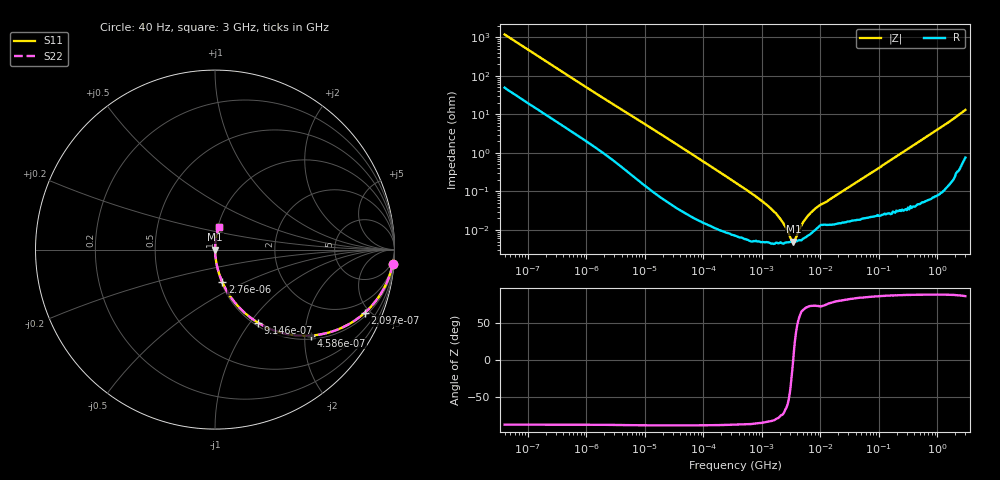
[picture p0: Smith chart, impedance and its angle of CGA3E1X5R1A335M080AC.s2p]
! S-parameter Generated by TDK Corporation
! Copyright(C) 2015 TDK Corporation.
! All Rights Reserved.
! TDK P/N: CGA3E1X5R1A335M080AC (Multilayer Ceramic Chip Capacitors)
! Property: C=3.3uF
! Size(LxWxT): 1.6x0.8x0.8mm, 0.063x0.031x0.031inches
! Model Type: s2p (Touchstone File Format Version 1.0)
! Frequency: DC=Yes Start=0.00004MHz Stop=3000MHz 396points Log-sweep
! Note: This model was converted from impedance.
! Model Generated on Jun. 23, 2015
! Hash(MD5):
! Port Assignments:
!  1 ---| |--- 2
! Applicable Conditions:
!  Temperature = 25 degC
!  DC Bias Voltage = 0 V
!  Small Signal Operation
! Terms and conditions regarding TDK Simulation Models
! (1)This simulation model is being provided solely for informational purposes. Please refer to the specifications of the products in terms of detailed characteristics of such products.
! (2)In no event shall TDK Corporation of any of its subsidiaries be liable for any loss or damage arising, directly or indirectly,
!  From any information contained in this simulation model, including, but not limited to loss or damages arising from any inaccuracies, omissions or errors in connection with such information.
! (3)Any and all copyrights on this simulation model are owned by TDK Corporation.
!  Duplication or redistribution of this simulation model without prior written permission from TDK Corporation is prohibited.
! (4)This simulation model is subject to any modification or change without any prior notice.
! (5)Neither TDK Corporation nor any of its subsidiaries shall make any warranty, express or implied,
!  Including but not limited to the correctness, implied warranties of merchantability and fitness for a particular purpose with respect to this simulation models.
! (6)The use of this simulation model shall be deemed to have consented to the terms and conditions hereof.
# MHz S MA R 50
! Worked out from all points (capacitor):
!   395 points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, 40 Hz to 3 GHz, reference 50 ohm
!   read as one part in series: C = 3.34 uF near 41.88 Hz
!   lowest |Z| = 4.99 mohm at 3.459 MHz (marker M1)
!   series resonance near 3.418 MHz, so ESL is about 650 pH
!   S11 on the Smith chart (normalised r, x): 40 Hz: 2, -24; 209.7 Hz: 1.19, -4.65; 458.6 Hz: 1.09, -2.15; 914.6 Hz: 1.04, -1.10; 2.76 kHz: 1.01, -0.38; 3 GHz: 1.02, +0.26
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4e-05  0.993 -4.8  0.08367 82.8  0.08367 82.8  0.993 -4.8
0.0001100992  0.9666 -12.7  0.2202 75.0  0.2202 75.0  0.9666 -12.7
0.000209705  0.9055 -22.9  0.3891 64.8  0.3891 64.8  0.9055 -22.9
0.0004585594  0.7187 -41.8  0.6669 45.9  0.6669 45.9  0.7187 -41.8
0.000834128  0.5054 -57.4  0.843 30.3  0.843 30.3  0.5054 -57.4
0.0009145504  0.4728 -59.5  0.8625 28.2  0.8625 28.2  0.4728 -59.5
0.001517294  0.3144 -69.5  0.9373 18.3  0.9373 18.3  0.3144 -69.5
0.002759985  0.1847 -77.3  0.9763 10.6  0.9763 10.6  0.1847 -77.3
0.006319477  0.08583 -83.4  0.9939 4.9  0.9939 4.9  0.08583 -83.4
0.01739424  0.03272 -86.8  0.9987 1.9  0.9987 1.9  0.03272 -86.8
0.3464102  0.00173 -87.6  0.9999 0.1  0.9999 0.1  0.00173 -87.6
1.315913  0.0004008 -83.3  1 0.0  1 0.0  0.0004008 -83.3
1.901634  0.0002278 -78.6  1 0.0  1 0.0  0.0002278 -78.6
2.748062  9.565e-05 -60.2  1 0.0  1 0.0  9.565e-05 -60.2
3.459106  4.994e-05 4.8  1 -0.0  1 -0.0  4.994e-05 4.8
4.354128  0.0001032 58.3  0.9999 -0.0  0.9999 -0.0  0.0001032 58.3
5.234209  0.000171 69.0  0.9999 -0.0  0.9999 -0.0  0.000171 69.0
7.22376  0.0003027 73.5  0.9999 -0.0  0.9999 -0.0  0.0003027 73.5
9.092863  0.0004083 73.4  0.9999 -0.0  0.9999 -0.0  0.0004083 73.4
150.6385  0.006187 87.1  0.9997 -0.4  0.9997 -0.4  0.006187 87.1
994.0817  0.03984 86.6  0.9984 -2.3  0.9984 -2.3  0.03984 86.6
3000  0.1286 79.3  0.9843 -7.4  0.9843 -7.4  0.1286 79.3
